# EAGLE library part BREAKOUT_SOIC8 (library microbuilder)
SOIC8 IC Breakout
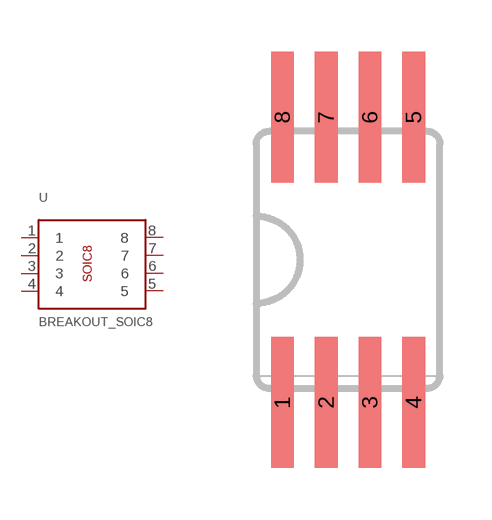
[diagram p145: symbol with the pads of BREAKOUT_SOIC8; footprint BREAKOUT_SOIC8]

Designator prefix U

## BREAKOUT_SOIC8  [BREAKOUT_SOIC8]
1  1
2  2
3  3
4  4
5  5
6  6
7  7
8  8

## Footprint BREAKOUT_SOIC8 (pad centres in mm)
smd 0.66 x 3.81: 1 -1.905,-4.14; 2 -0.635,-4.14; 3 0.635,-4.14; 4 1.905,-4.14; 5 1.905,4.14; 6 0.635,4.14; 7 -0.635,4.14; 8 -1.905,4.14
